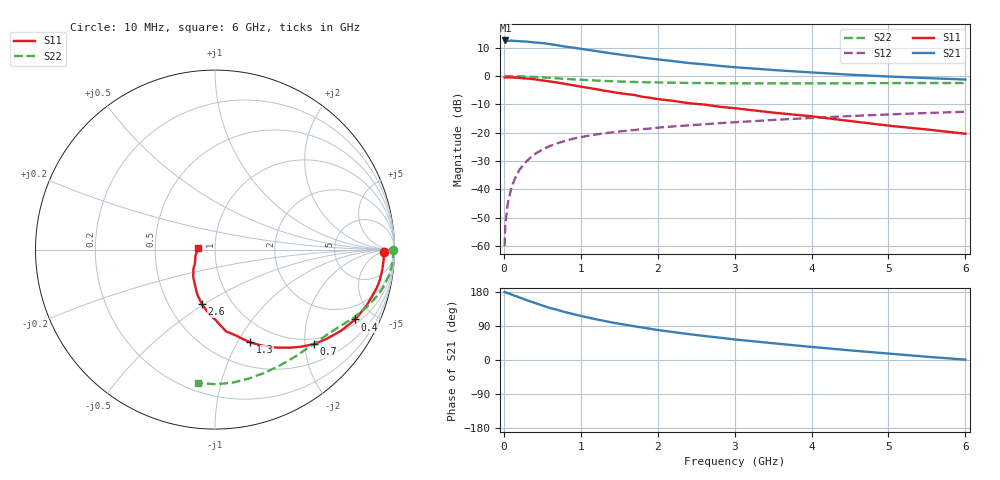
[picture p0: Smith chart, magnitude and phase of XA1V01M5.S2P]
! SIEMENS Discrete & RF Semiconductors
! BFY180
! Si NPN RF Bipolar Junction Transistor in MICRO-X
! VCE = 1 V  IC = 1.5 mA
! Common Emitter S-Parameters:  May  1997
# GHz  S  MA  R  50
!  f  S11  S21  S12  S22
! GHz  MAG  ANG  MAG  ANG  MAG  ANG  MAG  ANG
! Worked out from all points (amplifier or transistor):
!   36 points, 10 MHz to 6 GHz, reference 50 ohm
!   highest |S21| = 12.5 dB at 20 MHz (marker M1)
!   |S21| within 3 dB of that: start of sweep to 1.016 GHz
!   unconditionally stable (mu >= 1): 2.284 GHz to end of sweep
!   at 250 MHz: K = 0.13, MSG = 21.8 dB, |S12| = -31.4 dB
!   at 1.4 GHz: K = 0.75, MSG = 13.9 dB, |S12| = -19.9 dB
!   at 6 GHz: K = 1.15, MAG = 3.3 dB, |S12| = -12.6 dB
!   S11 on the Smith chart (normalised r, x): 10 MHz: 31, -6; 400 MHz: 1.20, -3.90; 700 MHz: 0.87, -2.20; 1.3 GHz: 0.76, -1.13; 2.6 GHz: 0.73, -0.49; 6 GHz: 0.83, +0.01
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0.01  0.9403 -0.7  4.169 179.4  0.001 75.6  0.9938 -0.2
0.02  0.9379 -1.4  4.218 178.5  0.0025 89.6  0.9999 -0.7
0.05  0.9415 -3.3  4.152 176.5  0.0055 88.9  0.9935 -1.6
0.1  0.939 -6.7  4.183 172.7  0.011 86.8  0.9909 -3.4
0.15  0.9341 -10.4  4.14 169.0  0.0162 83.8  0.9906 -5.0
0.3  0.9003 -20.3  4.023 157.7  0.0319 76.6  0.9728 -9.8
0.4  0.8725 -26.5  3.891 150.9  0.0418 73.0  0.9598 -12.8
0.5  0.8358 -32.7  3.789 143.9  0.0503 68.8  0.9429 -15.5
0.6  0.7976 -38.5  3.635 137.1  0.0584 65.6  0.923 -18.1
0.7  0.7623 -43.7  3.462 132.1  0.0653 62.0  0.9056 -20.5
0.8  0.722 -48.6  3.282 126.1  0.0719 59.7  0.8878 -22.6
0.9  0.6863 -52.8  3.154 121.4  0.0783 56.8  0.872 -24.7
1.1  0.6156 -61.5  2.867 111.8  0.0882 52.9  0.8424 -28.2
1.3  0.5513 -69.3  2.611 103.4  0.0971 49.4  0.8176 -31.5
1.5  0.4975 -75.6  2.394 95.6  0.1049 46.7  0.7972 -34.6
1.7  0.4605 -82.2  2.207 88.9  0.1117 44.6  0.7821 -37.5
2.2  0.364 -94.8  1.825 73.8  0.1289 39.9  0.7594 -44.6
2.6  0.3133 -103.4  1.605 63.5  0.1405 37.1  0.7481 -49.9
3.5  0.2256 -119.8  1.271 44.2  0.1676 30.6  0.7399 -61.9
4.5  0.1605 -138.4  1.052 25.4  0.1961 23.0  0.7433 -75.5
5.5  0.1139 -162.3  0.916 8.6  0.2222 14.7  0.7499 -90.0
6  0.0958 176.0  0.865 0.9  0.2338 10.3  0.7489 -97.4
